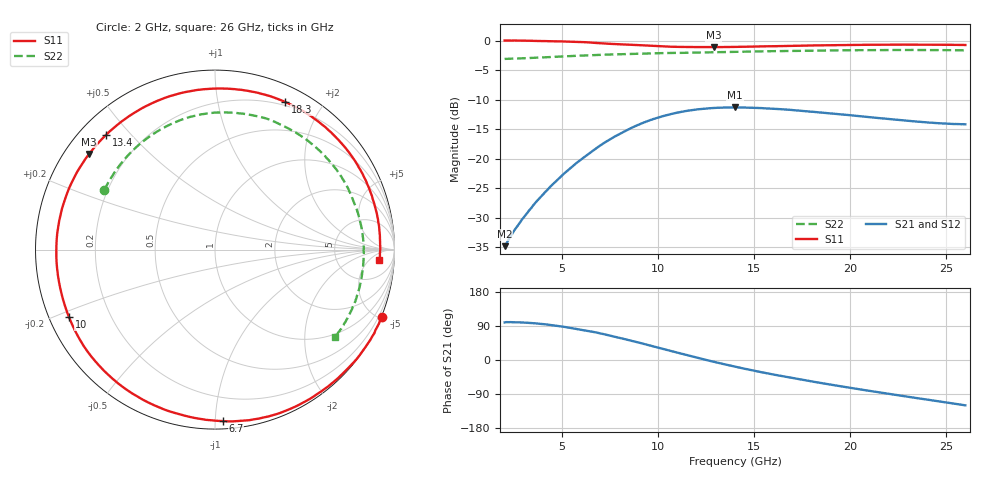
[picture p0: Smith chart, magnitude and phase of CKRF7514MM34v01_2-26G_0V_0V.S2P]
! CHUO DENSHI KOGYO Co.,Ltd.
! 30. May 2016
! CKRF7514MM34
! N-channel HJ-FET
! Vds = 0 V Vgs = 0 V
# Hz S  MA  R 50
!  f  S11  S21  S12  S22
!  Hz  MAG  ANG  MAG  ANG  MAG  ANG  MAG  ANG
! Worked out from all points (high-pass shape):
!   241 points, 2 GHz to 26 GHz, reference 50 ohm
!   highest |S21| = -11.31 dB at 14 GHz (marker M1); lowest = -34.8 dB at 2 GHz (marker M2)
!   |S21| within 3 dB of the highest: 8.927 GHz to end of sweep
!   lowest |S11| = -1.1 dB at 12.9 GHz (marker M3), VSWR 15.77, Z = 3.53 + j16.7 ohm
!   |S11| at or under -10 dB: nowhere
!   |S22| runs from -3.1 to -1.6 dB; largest |S21 - S12| = 0.00092
!   S11 on the Smith chart (normalised r, x): 2 GHz: -0.03, -5.11; 6.7 GHz: 0.05, -1.04; 10 GHz: 0.06, -0.22; 13.4 GHz: 0.07, +0.43; 18.3 GHz: 0.16, +1.57; 26 GHz: 15, -11
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2e9  1.002 -22.1  0.01819 99.2  0.01814 100.3  0.6998 151.7
2.9e9  0.999 -32.6  0.03045 98.9  0.03054 99.2  0.7077 140.0
4.1e9  0.9905 -47.7  0.05203 94.3  0.05203 94.4  0.7222 125.4
6e9  0.9726 -75.6  0.09901 79.7  0.09909 79.8  0.7471 104.8
6.7e9  0.9563 -87.5  0.1201 73.3  0.1199 73.3  0.755 98.0
7.6e9  0.937 -104.0  0.1495 63.0  0.1496 63.1  0.7637 89.7
8.4e9  0.9246 -119.9  0.1755 53.3  0.1758 53.4  0.7689 82.9
9.1e9  0.9134 -134.8  0.1976 44.5  0.1981 44.5  0.7741 77.3
1e10  0.8964 -155.1  0.2231 32.5  0.2233 32.6  0.7821 70.5
1.07e10  0.8869 -170.7  0.2396 23.3  0.2394 23.3  0.7859 65.1
1.14e10  0.8836 173.8  0.2526 14.1  0.2527 14.2  0.788 60.2
1.21e10  0.8816 158.9  0.2623 5.1  0.2623 5.2  0.7923 55.3
1.29e10  0.8807 142.8  0.2692 -4.8  0.2691 -4.7  0.7971 49.7
1.34e10  0.8814 133.4  0.271 -10.7  0.2713 -10.6  0.8003 46.3
1.4e10  0.8843 122.7  0.2719 -17.5  0.2719 -17.5  0.8028 42.3
1.57e10  0.895 96.4  0.2663 -35.4  0.2665 -35.3  0.8119 30.6
1.8e10  0.9092 67.8  0.2499 -56.6  0.2498 -56.5  0.8209 14.9
1.83e10  0.911 64.5  0.2475 -59.1  0.2476 -59.1  0.8223 12.9
2.02e10  0.9191 45.3  0.2315 -75.0  0.2314 -74.9  0.8275 -0.2
2.2e10  0.9237 28.8  0.2168 -89.2  0.2167 -89.2  0.8318 -12.0
2.42e10  0.9237 10.4  0.2021 -106.1  0.2019 -106.0  0.8309 -25.7
2.6e10  0.9173 -3.7  0.1954 -119.7  0.1957 -119.6  0.8282 -36.2
